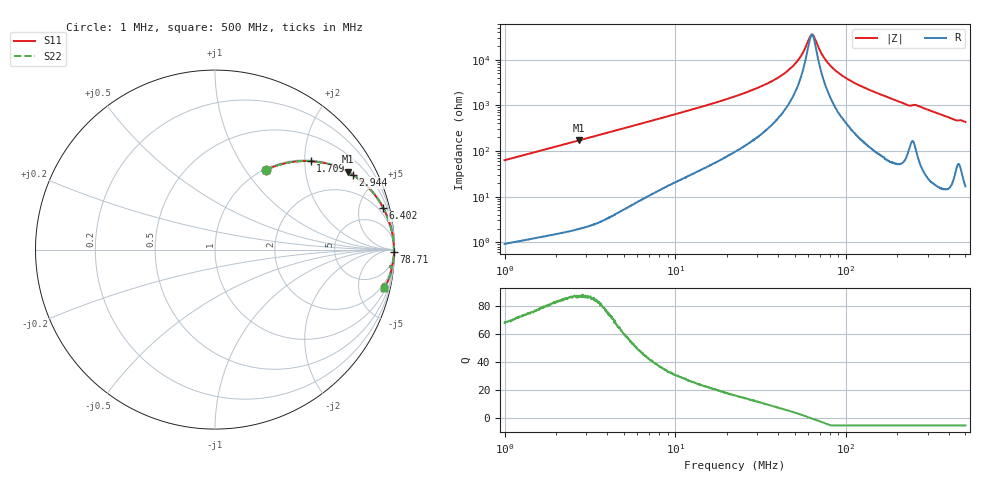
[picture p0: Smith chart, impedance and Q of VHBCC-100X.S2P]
!s-Parameter Generated by FASTRON Sdn. Bhd.
!FASTRON P/N : VHBCC-100X
!Keysight Technologies,E4991B,MY54100416,A.01.15
!Date: Mon Mar 16 11:56:40 2026
!Version  : Rev00 Mon Mar 16 11:56:40 2026
!Data & Calibration Information:
!PortZ  Port1:50+j0  Port2:50+j0
!When reading, reference impedance value at option line is always used.
! Remarks : This data is being provided solely for informational purposes.
!Freq	S11	S21	S12	S22
# Hz S dB R 50
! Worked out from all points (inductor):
!   1601 points, 1 MHz to 500 MHz, reference 50 ohm
!   read as one part in series: L = 9.95 uH near 1.032 MHz
!   highest Q = 87.2 at 2.713 MHz (marker M1), where L = 9.94 uH
!   self-resonance near 63.08 MHz
!   S11 on the Smith chart (normalised r, x): 1 MHz: 1.02, +1.25; 1.709 MHz: 1.03, +2.14; 2.944 MHz: 1.04, +3.68; 6.402 MHz: 1.18, +8.07; 78.71 MHz: open; 500 MHz: 1.33, -8.62
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1000000  -5.55 57.3  -1.50 -31.8  -1.50 -31.8  -5.55 57.3
1709174  -2.79 42.8  -3.36 -46.5  -3.36 -46.5  -2.79 42.8
2713451  -1.34 30.4  -5.92 -59.0  -5.92 -59.0  -1.34 30.4
2820919  -1.26 29.4  -6.17 -59.9  -6.17 -59.9  -1.26 29.4
2944056  -1.17 28.4  -6.46 -61.0  -6.46 -61.0  -1.17 28.4
6402024  -0.30 13.8  -12.42 -74.9  -12.42 -74.9  -0.30 13.8
7957584  -0.21 11.2  -14.26 -77.3  -14.26 -77.3  -0.21 11.2
2.236068e7  -0.05 3.6  -23.95 -82.9  -23.95 -82.9  -0.05 3.6
3.388275e7  -0.03 2.0  -29.26 -82.5  -29.26 -82.5  -0.03 2.0
4.464218e7  -0.03 1.1  -34.60 -79.5  -34.60 -79.5  -0.03 1.1
5.316844e7  -0.03 0.5  -40.48 -71.8  -40.48 -71.8  -0.03 0.5
6.114779e7  -0.02 0.1  -49.68 -30.8  -49.68 -30.8  -0.02 0.1
6.307767e7  -0.02 0.0  -50.94 -1.2  -50.94 -1.2  -0.02 0.0
6.506845e7  -0.02 -0.1  -49.91 29.2  -49.91 29.2  -0.02 -0.1
7.170375e7  -0.02 -0.4  -42.75 67.4  -42.75 67.4  -0.02 -0.4
7.870937e7  -0.02 -0.7  -38.37 76.2  -38.37 76.2  -0.02 -0.7
9.01709e7  -0.02 -1.1  -34.23 81.3  -34.23 81.3  -0.02 -1.1
1.057371e8  -0.03 -1.6  -30.83 83.2  -30.83 83.2  -0.03 -1.6
1.77937e8  -0.04 -3.9  -23.42 83.8  -23.42 83.8  -0.04 -3.9
2.290403e8  -0.11 -5.6  -20.23 79.6  -20.23 79.6  -0.11 -5.6
2.573461e8  -0.13 -5.6  -20.17 78.7  -20.17 78.7  -0.13 -5.6
5e8  -0.30 -12.9  -12.99 74.8  -12.99 74.8  -0.30 -12.9
